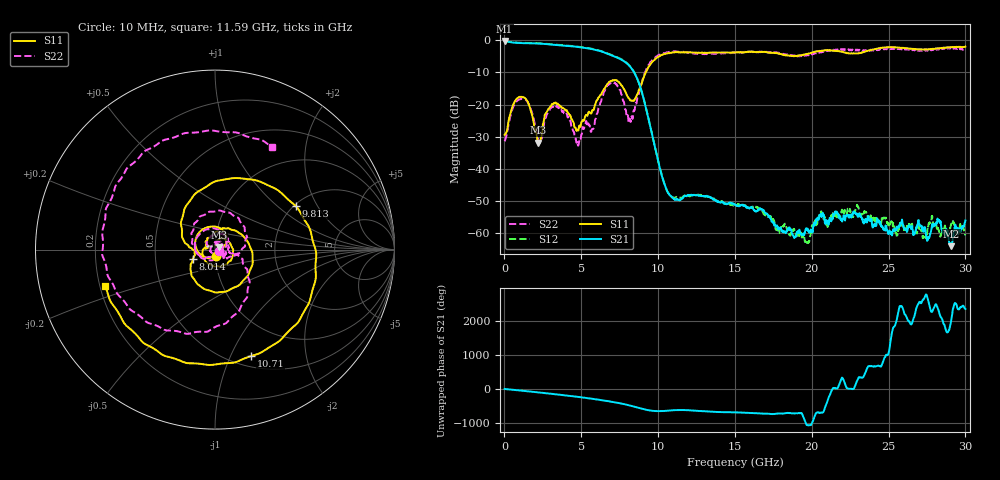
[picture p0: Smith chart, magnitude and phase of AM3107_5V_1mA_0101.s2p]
# Hz S DB R 50.0
!freq dBS11 angS11 dBS21 angS21 dBS12 angS12 dBS22 angS22
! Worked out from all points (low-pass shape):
!   1601 points, 10 MHz to 30 GHz, reference 50 ohm
!   highest |S21| = -0.20 dB at 10 MHz (marker M1); lowest = -64.1 dB at 29.08 GHz (marker M2)
!   |S21| within 3 dB of the highest: start of sweep to 6.09 GHz
!   lowest |S11| = -31.9 dB at 2.184 GHz (marker M3), VSWR 1.05, Z = 52.1 + j1.55 ohm
!   |S11| at or under -10 dB: start of sweep to 9.198 GHz
!   |S22| runs from -32.8 to -2.2 dB; largest |S21 - S12| = 0.014
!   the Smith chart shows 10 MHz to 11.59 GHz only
!   S11 on the Smith chart (normalised r, x): 10 MHz: 1.01, -0.07; 8.014 GHz: 0.78, -0.08; 9.813 GHz: 2.04, +1.34; 10.71 GHz: 0.61, -1.20; 11.59 GHz: 0.22, -0.15
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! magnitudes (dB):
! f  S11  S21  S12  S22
! 10 MHz  -29.4  -0.2  -0.1  -31.4
! 1.135 GHz  -17.6  -0.9  -0.8  -18.2
! 2.184 GHz  -31.9  -1.0  -0.9  -30.7
! 3.309 GHz  -19.4  -1.5  -1.4  -20.3
! 5.015 GHz  -25.5  -2.3  -2.2  -29.4
! 5.727 GHz  -21.7  -2.8  -2.7  -27.6
! 6.945 GHz  -12.6  -4.7  -4.6  -13.2
! 8.014 GHz  -17.5  -7.4  -7.3  -23.3
! 8.838 GHz  -14.5  -14.6  -14.4  -15.5
! 9.813 GHz  -5.8  -33.7  -33.6  -5.4
! 10.02 GHz  -5.2  -37.9  -37.8  -4.7
! 10.71 GHz  -4.1  -47.9  -47.8  -3.6
! 11.59 GHz  -3.8  -49.2  -48.9  -3.7
! 15.01 GHz  -3.8  -51.1  -51.5  -3.8
! 19.69 GHz  -4.2  -58.7  -63.1  -4.7
! 20.01 GHz  -3.9  -59.6  -57.7  -4.4
! 22.82 GHz  -4.1  -53.7  -53.1  -3.2
! 25.01 GHz  -2.2  -59.8  -58.0  -2.7
! 27.58 GHz  -2.8  -61.2  -58.0  -2.9
! 28.26 GHz  -2.5  -55.9  -59.0  -2.9
! 29.08 GHz  -2.2  -64.1  -57.0  -2.5
! 30 GHz  -2.0  -56.1  -60.3  -2.4
